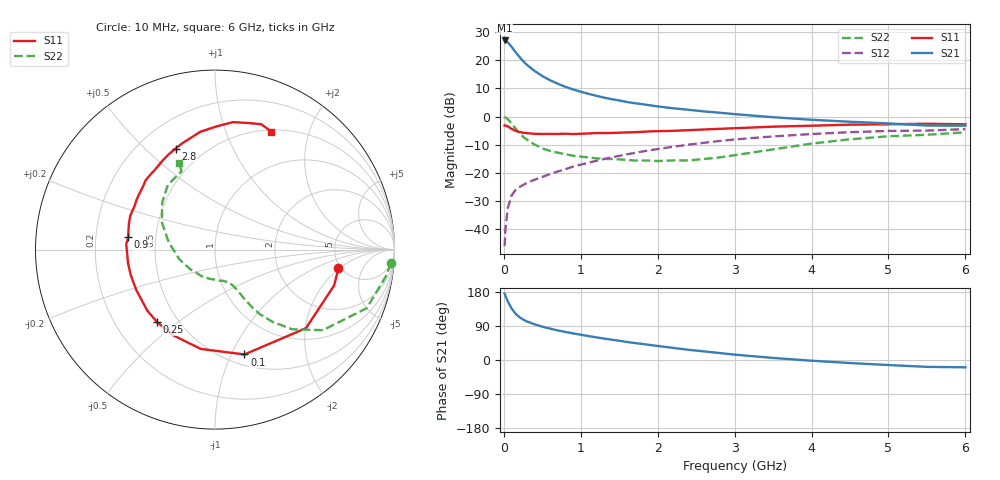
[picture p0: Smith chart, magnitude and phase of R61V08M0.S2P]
! SIEMENS Small Signal Semiconductors
! BFR193
! Si NPN RF Bipolar Junction Transistor in SOT23
! VCE = 1 V  IC = 8 mA
! Common Emitter S-Parameters:  May  1996
# GHz  S  MA  R  50
!  f  S11  S21  S12  S22
! GHz  MAG  ANG  MAG  ANG  MAG  ANG  MAG  ANG
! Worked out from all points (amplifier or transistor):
!   36 points, 10 MHz to 6 GHz, reference 50 ohm
!   highest |S21| = 27.0 dB at 10 MHz (marker M1)
!   |S21| within 3 dB of that: start of sweep to 120.8 MHz
!   unconditionally stable (mu >= 1): 756.3 MHz to 2.19 GHz
!   at 250 MHz: K = 0.58, MSG = 22.0 dB, |S12| = -24.3 dB
!   at 1.4 GHz: K = 1.06, MAG = 8.8 dB, |S12| = -14.5 dB
!   at 6 GHz: K = 0.98, MSG = 0.6 dB, |S12| = -4.5 dB
!   S11 on the Smith chart (normalised r, x): 10 MHz: 4.75, -1.94; 100 MHz: 0.61, -1.12; 250 MHz: 0.38, -0.42; 900 MHz: 0.35, +0.06; 2.8 GHz: 0.35, +0.62; 6 GHz: 0.52, +1.46
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0.01  0.6958 -8.7  22.41 175.0  0.005 84.0  0.9821 -4.5
0.02  0.6928 -16.8  21.96 169.7  0.0099 81.9  0.9642 -8.8
0.05  0.6697 -40.8  20.92 155.3  0.0231 72.3  0.9061 -21.1
0.1  0.6069 -74.3  17.37 136.3  0.0394 60.4  0.7508 -36.7
0.15  0.5589 -98.2  13.97 122.8  0.0494 53.6  0.6179 -45.9
0.2  0.5313 -115.4  11.58 113.5  0.0557 51.2  0.5137 -51.5
0.25  0.5166 -128.6  9.66 106.8  0.061 50.0  0.4385 -55.2
0.3  0.5079 -137.9  8.272 101.7  0.0663 49.7  0.3894 -57.0
0.4  0.493 -152.9  6.448 94.2  0.0756 51.4  0.3183 -59.2
0.5  0.4903 -163.1  5.224 87.9  0.085 53.5  0.2717 -60.7
0.6  0.4906 -171.1  4.412 82.8  0.0952 54.9  0.2451 -61.9
0.7  0.4899 -177.7  3.828 78.1  0.1058 56.2  0.2284 -63.2
0.9  0.4887 171.8  3.027 70.2  0.1286 57.6  0.2015 -66.3
1.1  0.5013 163.0  2.53 63.2  0.1517 58.1  0.1877 -71.6
1.3  0.5087 155.1  2.172 56.6  0.1761 57.5  0.1772 -77.3
1.6  0.5224 144.5  1.809 47.6  0.2133 55.9  0.1698 -88.7
2.2  0.5571 126.8  1.401 32.0  0.2908 50.1  0.1662 -117.6
2.8  0.6044 111.3  1.17 18.5  0.3677 42.0  0.1876 -154.7
3.5  0.6611 97.2  0.972 5.4  0.4438 31.0  0.2612 170.9
4.5  0.7171 82.0  0.808 -8.0  0.5279 15.8  0.3943 138.3
5.5  0.7446 69.8  0.691 -18.1  0.5633 1.0  0.4747 113.1
6  0.729 64.5  0.689 -19.3  0.5978 -3.5  0.5243 112.5
